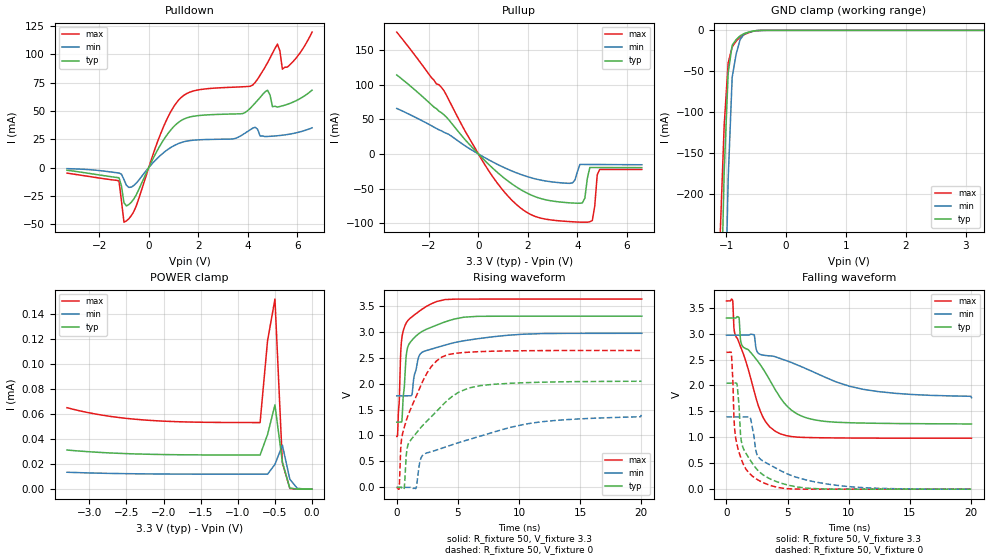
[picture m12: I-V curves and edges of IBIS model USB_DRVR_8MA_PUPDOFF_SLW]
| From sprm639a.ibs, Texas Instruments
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|   Model Cell USB_DRVR_8MA_PUPDOFF_SLW
|USB_DRVR_8MA_PUPDOFF_SLW
[Model]   USB_DRVR_8MA_PUPDOFF_SLW
Model_type   I/O
Polarity   Non-Inverting
Enable   Active-Low
Vinl =  0.8
Vinh =  2
Cref =  15.0000pF
Rref =  100.0000M
Vref =  0V
Vmeas =  1.65
C_comp   5.34973p   4.565931p   6.027791p
[Model Spec]
Vinl   0.8   0.8   0.8
Vinh   2   2   2
[Temperature Range]   25   155   -40
[Voltage Range]   3.3   2.97   3.63
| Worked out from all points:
|   slope of the pulldown table from 0 to 0.495 V, typ, clamps not added: 23.8 ohm
|   slope of the pullup table from 0 to 0.495 V, typ, clamps not added: 27.8 ohm
|   GND clamp passes 1 mA (typ) near -0.55 V on its own axis
|   rising waveform, R_fixture 50, V_fixture 3.3: 20-80 % time 953ps typ, 2.4ns min, 493ps max; typ from 1.26 V to 3.3 V
|   rising waveform, R_fixture 50, V_fixture 0: 20-80 % time 3.24ns typ, 6.93ns min, 1.98ns max; typ from 0 V to 2.04 V
|   falling waveform, R_fixture 50, V_fixture 3.3: 20-80 % time 3.57ns typ, 7.38ns min, 2.14ns max; typ from 3.3 V to 1.26 V
|   falling waveform, R_fixture 50, V_fixture 0: 20-80 % time 1.37ns typ, 2.98ns min, 774ps max; typ from 2.04 V to 0 V
| Nom Voltages:
|   BIASFET=3.3, VDD=1.2, VDDS=3.3, VSS=0
| Min Voltages:
|   BIASFET=2.97, VDD=1.08, VDDS=2.97, VSS=0
| Max Voltages:
|   BIASFET=3.63, VDD=1.32, VDDS=3.63, VSS=0
[POWER_clamp]
|   voltage   I(typ)   I(min)   I(max)
-3.3V     31.22uA    13.5uA     64.95uA
-2.8V     29.13uA    12.67uA    58.77uA
-2.3V     27.98uA    12.22uA    55.36uA
-1.7V     27.4uA     12.01uA    53.62uA
-700mV    27.24uA    11.95uA    53.12uA
-600mV    43.52uA    11.94uA    118.2uA
-500mV    67.21uA    19.79uA    151.6uA
-400mV    21.58uA    35.11uA    21.1uA
-300mV    927.4nA    7.959uA    611.4nA
-200mV    28.93nA    716.3nA    11.51nA
0V        696.9pA    39.48nA    568.3pA
[Pulldown]
|   voltage   I(typ)   I(min)   I(max)
-3.3V     -2.325mA   -885.1uA   -4.829mA
-1.2V     -8.9mA     -4.742mA   -11.78mA
-1V       -30.94mA   -10.56mA   -48.07mA
-900mV    -33.77mA   -15.53mA   -46.9mA
-500mV    -23.82mA   -13.61mA   -33.55mA
600mV     24.46mA    13.16mA    36.18mA
1.3V      41.39mA    22.04mA    61.62mA
4.2V      54.57mA    34.77mA    72.77mA
4.8V      68.22mA    27.49mA    92.41mA
5.2V      53.41mA    28.11mA    108.9mA
5.4V      54.46mA    28.58mA    86.79mA
6.6V      68.25mA    35.07mA    119.5mA
[Pullup]
|   voltage   I(typ)   I(min)   I(max)
-3.3V     114.4mA    65.88mA    176.4mA
-1.4V     56.91mA    31.53mA    92.06mA
700mV     -24.56mA   -13.78mA   -39.08mA
2V        -57.24mA   -33.05mA   -85.4mA
3.8V      -70.97mA   -41.82mA   -98.09mA
4.2V      -70.71mA   -15.14mA   -98.64mA
4.5V      -19.61mA   -15.2mA    -98.06mA
4.6V      -19.61mA   -15.22mA   -96.39mA
4.7V      -19.61mA   -15.23mA   -75.23mA
4.8V      -19.61mA   -15.26mA   -30.07mA
4.9V      -19.62mA   -15.28mA   -22.42mA
6.6V      -19.78mA   -15.6mA    -22.44mA
[GND_clamp]
|   voltage   I(typ)   I(min)   I(max)
-3.3V     -16.36A    -15.08A    -17.18A
-1.1V     -382.1mA   -717.8mA   -250.1mA
-1.033V   -173.3mA   -402.2mA   -116.4mA
-966.7mV  -52.02mA   -182.1mA   -39.81mA
-900mV    -18.21mA   -57.43mA   -20.34mA
-833.3mV  -11.36mA   -28.88mA   -13.17mA
-766.7mV  -6.618mA   -11.27mA   -8.134mA
-700mV    -3.983mA   -4.59mA    -5.247mA
-500mV    -328.3uA   -481.4uA   -374.5uA
-366.7mV  -15.94uA   -50.74uA   -14.83uA
3.3V      696.9pA    15.85uA    426.1pA
[Ramp]
| variable   typ   min   max
dV/dt_f  1.2421653/3.5598598n 0.73476831/7.3439451n  1.6102559/2.1405336n
dV/dt_r  1.2473475/3.2240532n 0.85354234/6.8883736n   1.604522/1.9717405n
R_load = 50
[Rising Waveform]
R_fixture = 50
V_fixture = 3.3
V_fixture_min = 2.97
V_fixture_max = 3.63
|   time   V(typ)   V(min)   V(max)
0s        1.258V     1.765V     982.5mV
202.6ps   1.258V     1.765V     1.64V
335.7ps   1.256V     1.765V     2.643V
477ps     1.525V     1.765V     2.965V
906.4ps   2.71V      1.765V     3.215V
1.247ns   2.837V     1.791V     3.289V
1.806ns   2.963V     2.521V     3.389V
2.381ns   3.044V     2.634V     3.483V
6.491ns   3.297V     2.861V     3.63V
20.04ns   3.3V       2.97V      3.63V
[Rising Waveform]
R_fixture = 50
V_fixture = 0
V_fixture_min = 0
V_fixture_max = 0
|   time   V(typ)   V(min)   V(max)
0s        0V         0V         0V
195.1ps   0V         0V         -24.08mV
354.9ps   0V         0V         845.8mV
603.7ps   -24.96mV   0V         1.148V
894.4ps   801.8mV    0V         1.368V
1.575ns   1.041V     -15.88mV   1.745V
2.111ns   1.191V     617mV      2.037V
3.731ns   1.583V     757.2mV    2.517V
6.844ns   1.961V     988mV      2.617V
20.01ns   2.045V     1.397V     2.639V
[Falling Waveform]
R_fixture = 50
V_fixture = 3.3
V_fixture_min = 2.97
V_fixture_max = 3.63
|   time   V(typ)   V(min)   V(max)
0s        3.3V       2.97V      3.63V
508.4ps   3.3V       2.97V      3.644V
675.8ps   3.3V       2.97V      3.009V
1.032ns   3.304V     2.97V      2.822V
1.262ns   2.779V     2.97V      2.686V
2.242ns   2.563V     2.979V     1.903V
2.763ns   2.402V     2.6V       1.509V
3.97ns    1.927V     2.555V     1.119V
7.274ns   1.333V     2.243V     992.8mV
20.04ns   1.258V     1.765V     982.8mV
[Falling Waveform]
R_fixture = 50
V_fixture = 0
V_fixture_min = 0
V_fixture_max = 0
|   time   V(typ)   V(min)   V(max)
0s        2.045V     1.393V     2.639V
403.6ps   2.045V     1.393V     2.614V
511.9ps   2.045V     1.393V     2.187V
649.9ps   2.045V     1.393V     1.229V
896.7ps   1.964V     1.393V     825.1mV
1.28ns    858.3mV    1.393V     537.1mV
1.95ns    558.6mV    1.377V     287.8mV
2.666ns   338.9mV    603.7mV    165mV
8.298ns   2.125mV    96.69mV    0V
20.01ns   0V         0V         0V
